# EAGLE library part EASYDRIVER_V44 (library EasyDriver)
EasyDriver version 4.4 - http://www.schmalzhaus.com/EasyDriver
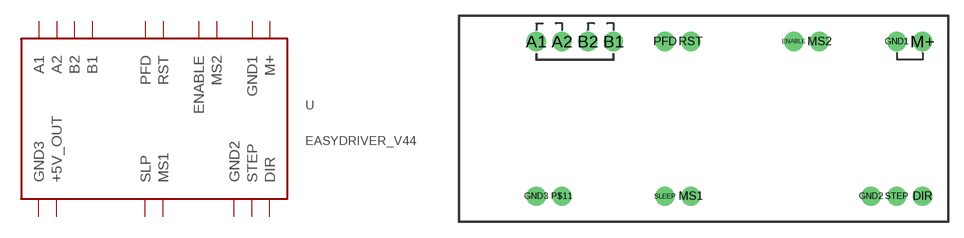
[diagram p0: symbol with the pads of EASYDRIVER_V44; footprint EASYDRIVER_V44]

Designator prefix -

## EASYDRIVER_V44  [EASYDRIVER_V44]
A1  A1
A2  A2
B1  B1
B2  B2
DIR  DIR
ENABLE  ENABLE
GND1  GND1
GND2  GND2
GND3  GND3
M+  M+
MS1  MS1
MS2  MS2
P$11  +5V_OUT
PFD  PFD
RST  RST
SLEEP  SLP
STEP  STEP

## Footprint EASYDRIVER_V44 (pad centres in mm)
drill 1.016 pad 1.88: A1 -16.51,7.62; A2 -13.97,7.62; B1 -8.89,7.62; B2 -11.43,7.62; DIR 21.59,-7.62; ENABLE 8.89,7.62; GND1 19.05,7.62; GND2 16.51,-7.62; GND3 -16.51,-7.62; M+ 21.59,7.62; MS1 -1.27,-7.62; MS2 11.43,7.62; P$11 -13.97,-7.62; PFD -3.81,7.62; RST -1.27,7.62; SLEEP -3.81,-7.62; STEP 19.05,-7.62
